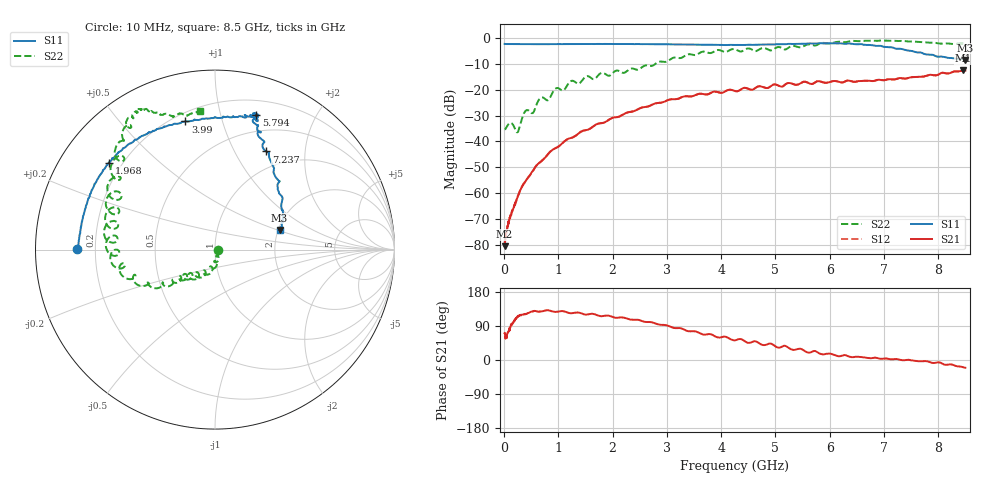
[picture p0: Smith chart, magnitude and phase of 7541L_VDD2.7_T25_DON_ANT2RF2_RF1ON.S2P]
!Agilent Technologies,E5071C,MY46417908,A.11.23
!Date: Wed Dec 09 17:17:15 2020
!Data & Calibration Information:
!Freq	S11:SOLT2(ON)	S21:SOLT2(ON)	S12:SOLT2(ON)	S22:SOLT2(ON)
!PortZ  Port1:50+j0  Port2:50+j0
!Above PortZ is port z conversion or system Z0 setting when saving the data.
!When reading, reference impedance value at option line is always used.
# Hz S dB R 50
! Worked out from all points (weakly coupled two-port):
!   1601 points, 10 MHz to 8.5 GHz, reference 50 ohm
!   highest |S21| = -12.58 dB at 8.463 GHz (marker M1); lowest = -80.5 dB at 10 MHz (marker M2)
!   lowest |S11| = -8.5 dB at 8.5 GHz (marker M3), VSWR 2.21, Z = 102 + j26 ohm
!   |S11| at or under -10 dB: nowhere
!   |S22| runs from -36.5 to -1.0 dB; largest |S21 - S12| = 0.0029
!   S11 on the Smith chart (normalised r, x): 10 MHz: 0.13, +0.00; 1.968 GHz: 0.15, +0.35; 3.99 GHz: 0.25, +0.77; 5.794 GHz: 0.33, +1.30; 7.237 GHz: 0.76, +1.35; 8.5 GHz: 2.03, +0.52
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1e7  -2.31 179.6  -80.51 70.7  -80.19 67.6  -35.35 -3.2
1.16125e8  -2.37 177.3  -69.07 85.9  -68.51 85.0  -32.82 -41.8
2.700062e8  -2.39 174.0  -60.53 117.1  -60.33 117.8  -35.51 -45.7
3.9205e8  -2.41 171.0  -55.52 120.4  -55.52 121.4  -28.29 -64.4
5.565438e8  -2.41 167.7  -50.56 129.4  -50.56 129.5  -28.12 -66.8
6.626688e8  -2.41 165.5  -48.05 127.9  -48.07 127.6  -23.35 -78.3
8.112438e8  -2.41 162.5  -44.87 131.3  -44.86 131.3  -24.04 -88.2
9.545125e8  -2.39 159.4  -42.54 126.8  -42.54 126.7  -19.50 -94.5
1.426769e9  -2.36 150.4  -36.13 122.8  -36.13 122.8  -16.74 -111.4
1.968006e9  -2.34 140.7  -31.17 115.4  -31.17 115.4  -14.28 -130.5
2.843538e9  -2.42 126.1  -25.13 93.8  -25.13 93.9  -9.32 -143.4
3.602331e9  -2.62 112.1  -21.57 71.0  -21.57 71.0  -5.81 -161.4
3.989688e9  -2.70 103.0  -21.21 59.5  -21.22 59.6  -4.82 -178.6
4.255e9  -2.72 95.8  -20.52 52.0  -20.53 51.9  -4.40 174.8
5.226044e9  -2.32 76.9  -17.49 33.6  -17.49 33.7  -3.99 153.6
5.671769e9  -2.18 73.9  -17.82 21.6  -17.76 21.6  -2.62 135.0
5.793812e9  -2.09 72.9  -16.71 18.4  -16.71 18.7  -2.42 137.0
6.202394e9  -2.09 72.9  -17.16 10.5  -17.16 10.8  -1.43 125.3
7.088538e9  -3.56 65.9  -15.95 2.8  -16.00 2.7  -1.10 118.0
7.237112e9  -4.20 62.5  -15.80 2.6  -15.81 2.6  -1.17 117.0
8.462856e9  -8.31 18.1  -12.58 -19.2  -12.65 -19.3  -2.22 97.2
8.5e9  -8.49 17.0  -12.60 -20.5  -12.69 -20.4  -2.19 96.1
